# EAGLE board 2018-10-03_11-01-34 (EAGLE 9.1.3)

Size 160 x 100 mm. Coordinates in mm from the lower left corner, seen from the top.
Outline: 0,0 160,0 160,100 0,100 0,0
Copper layers (1*16): Top 0.035mm / dielectric 1.5mm / Bottom 0.035mm
Design rules "default": minimum track width 6mil, minimum drill 0.35mm, track to track 6mil, track to pad 6mil, pad to pad 6mil, via to via 6mil, smd to smd 6mil, copper to edge 40mil, drill to drill 6mil, minimum pad ring 10mil, minimum via ring 8mil, stop-mask expansion 4mil, vias tented up to drill 0mil, thermal gap 10mil

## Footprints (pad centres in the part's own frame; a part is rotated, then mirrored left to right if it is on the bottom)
0603 = drill 0: 1 -0.699,0; 2 0.699,0
1812 = drill 0: 1 -2.273,0; 2 2.273,0
CAPSMT_62_C10 = drill 0: 1 -2.273,0; 2 2.273,0
SM_RADIAL_J16 = drill 0: 1 -6.566,0; 2 6.566,0
1210_270 = drill 0: 1 -1.45,0; 2 1.45,0
0402 = drill 0: 1 -0.419,0; 2 0.419,0
SOD-323 = drill 0: 1 -1.1,0; 2 1.1,0
WB_GND = drill 0: 1 0,0
WB_CURRENT_LOAD = drill 0: 1 0,0; 2 0,0
MSS1210 = drill 0: 1 -4.763,0; 2 4.763,0
TRANS_NEXFET_Q5B = drill 0: 1 -2.77,1.905; 2 -2.77,0.635; 3 -2.77,-0.635; 4 -2.77,-1.905; 5 2.77,-1.905; 6 2.77,-0.635; 7 2.77,0.635; 8 2.77,1.905; 9 1.16,0
DNH0008A = drill 0: 1 -1.625,0.975; 2 -1.625,0.325; 3 -1.625,-0.325; 4 -1.625,-0.975; 5 1.385,-0.975; 6 1.385,-0.325; 7 1.385,0.325; 8 1.385,0.975; 9 0.205,0
0201 = drill 0: 1 -0.292,0; 2 0.292,0
2512 = drill 0: 1 -2.248,0; 2 2.248,0
1210 = drill 0: 1 -1.499,0; 2 1.499,0
MXA20A = drill 0: 1 -2.845,2.925; 2 -2.845,2.275; 3 -2.845,1.625; 4 -2.845,0.975; 5 -2.845,0.325; 6 -2.845,-0.325; 7 -2.845,-0.975; 8 -2.845,-1.625; 9 -2.845,-2.275; 10 -2.845,-2.925; 11 2.845,-2.925; 12 2.845,-2.275; 13 2.845,-1.625; 14 2.845,-0.975; 15 2.845,-0.325; 16 2.845,0.325; 17 2.845,0.975; 18 2.845,1.625; 19 2.845,2.275; 20 2.845,2.925; 21 0,0
WB_BATTERY = drill 0: 1 0,0; 2 0,0

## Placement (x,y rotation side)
CBST  330nF  [0603]  not placed on the board
CCOMP  27nF  [1812]  not placed on the board
CCOMP2  1.5nF  [0603]  not placed on the board
CIN  270uF  [CAPSMT_62_C10]  not placed on the board
COUT  470uF  [SM_RADIAL_J16]  not placed on the board
COUT_2  470uF  [SM_RADIAL_J16]  not placed on the board
COUT_3  470uF  [SM_RADIAL_J16]  not placed on the board
COUT_4  470uF  [SM_RADIAL_J16]  not placed on the board
COUTX  10uF  [1210_270]  not placed on the board
COUTX_2  10uF  [1210_270]  not placed on the board
COUTX_3  10uF  [1210_270]  not placed on the board
COUTX_4  10uF  [1210_270]  not placed on the board
CRES  470nF  [0603]  not placed on the board
CSS  220nF  [0402]  not placed on the board
CVCC  4.7uF  [0603]  not placed on the board
CVIN  470nF  [0603]  not placed on the board
DBST  540mV  [SOD-323]  not placed on the board
GND1  WB_GND  [WB_GND]  not placed on the board
GND2  WB_GND  [WB_GND]  not placed on the board
GND3  WB_GND  [WB_GND]  not placed on the board
GND4  WB_GND  [WB_GND]  not placed on the board
GND5  WB_GND  [WB_GND]  not placed on the board
IOUT  WB_CURRENT_LOAD  [WB_CURRENT_LOAD]  not placed on the board
L1  68uH  [MSS1210]  not placed on the board
M1  60V  [TRANS_NEXFET_Q5B]  not placed on the board
M2  60V  [DNH0008A]  not placed on the board
RCOMP  36.5k  [0201]  not placed on the board
RFBB  1.6k  [0603]  not placed on the board
RFBT  46.4k  [0402]  not placed on the board
RSENSE  4m  [2512]  not placed on the board
RSLOPE  301k  [0402]  not placed on the board
RT  162k  [0201]  not placed on the board
RUVB  8.25k  [0402]  not placed on the board
RUVT  51.1k  [0402]  not placed on the board
RVIN  2.74  [1210]  not placed on the board
U1  LM5122MH/NOPB  [MXA20A]  not placed on the board
VIN  WB_BATTERY  [WB_BATTERY]  not placed on the board

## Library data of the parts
CBST = AcceleratedDesigns_Lib; CAP: 3.3E-7; DATASHEET_URL: https://product.tdk.com/en/search/capacitor/ceramic/mlcc/info?part%5Fno%3DC1608X5R1H334K080AB; ESR: 0.016574; IRMS: 1.28367; MANUFACTURER_NAME: TDK; MANUFACTURER_PART_NUMBER: C1608X5R1H334K080AB; VDC: 50.0; VENDOR: TDK
CCOMP = AcceleratedDesigns_Lib; CAP: 2.7E-8; DATASHEET_URL: http://www.kemet.com/docfinder?Partnumber%3DC1812C273J5GACTU; ESR: 0.0; IRMS: 0.0; MANUFACTURER_NAME: Kemet; MANUFACTURER_PART_NUMBER: C1812C273J5GACTU; VDC: 50.0; VENDOR: Kemet
CCOMP2 = AcceleratedDesigns_Lib; CAP: 1.5E-9; DATASHEET_URL: http://www.murata.com/products/catalog/pdf/c03e.pdf; ESR: 0.0; IRMS: 0.0; MANUFACTURER_NAME: MuRata; MANUFACTURER_PART_NUMBER: GCM1885C1H152JA16D; VDC: 50.0; VENDOR: MuRata
CIN = AcceleratedDesigns_Lib; CAP: 2.7E-4; DATASHEET_URL: %20; ESR: 0.008; IRMS: 5.8; MANUFACTURER_NAME: Panasonic; MANUFACTURER_PART_NUMBER: 16SVPG270M; VDC: 16.0; VENDOR: Panasonic
COUT COUT_2-COUT_4 = AcceleratedDesigns_Lib; CAP: 4.7E-4; DATASHEET_URL: http://www.panasonic.com/industrial/components/pdf/smt%5Faec%5F050505.pdf; ESR: 0.082; IRMS: 1.41; MANUFACTURER_NAME: Panasonic; MANUFACTURER_PART_NUMBER: EEV-FK1J471M; VDC: 63.0; VENDOR: Panasonic
COUTX COUTX_2-COUTX_4 = AcceleratedDesigns_Lib; CAP: 1.0E-5; DATASHEET_URL: http://www.samsungsem.com/kr/support/product%2Dsearch/mlcc/%5F%5FicsFiles/afieldfile/2016/08/18/S%5FCL32B106KBJNNWE.pdf; ESR: 0.005; IRMS: 0.0; MANUFACTURER_NAME: Samsung Electro-Mechanics; MANUFACTURER_PART_NUMBER: CL32B106KBJNNWE; VDC: 50.0; VENDOR: Samsung Electro-Mechanics
CRES = AcceleratedDesigns_Lib; CAP: 4.7E-7; ESR: 0.0; IRMS: 0.0; MANUFACTURER_NAME: MuRata; MANUFACTURER_PART_NUMBER: GRM188R71E474KA12D; VDC: 25.0; VENDOR: MuRata
CSS = AcceleratedDesigns_Lib; CAP: 2.2E-7; ESR: 0.0; IRMS: 0.0; MANUFACTURER_NAME: MuRata; MANUFACTURER_PART_NUMBER: GRM155R61A224KE19D; VDC: 10.0; VENDOR: MuRata
CVCC = AcceleratedDesigns_Lib; CAP: 4.7E-6; DATASHEET_URL: https://product.tdk.com/en/search/capacitor/ceramic/mlcc/info?part%5Fno%3DC1608X6S1C475K080AC; ESR: 0.003728; IRMS: 2.69359; MANUFACTURER_NAME: TDK; MANUFACTURER_PART_NUMBER: C1608X6S1C475K080AC; VDC: 16.0; VENDOR: TDK
CVIN = AcceleratedDesigns_Lib; CAP: 4.7E-7; ESR: 0.0; IRMS: 0.0; MANUFACTURER_NAME: MuRata; MANUFACTURER_PART_NUMBER: GRM188R61C474KA93D; VDC: 16.0; VENDOR: MuRata
DBST = AcceleratedDesigns_Lib; DATASHEET_URL: http://www.torexsemi.com/products/schottky%5Fbarrier%5Fdiodes/data/XBS104S13.pdf; IO: 1.0; MANUFACTURER_NAME: Torex USA Corporation; MANUFACTURER_PART_NUMBER: XBS104S13R-G; VENDOR: Torex USA Corporation; VFATIO: 0.54; VRRM: 40.0
GND1-GND5 = AcceleratedDesigns_Lib; MANUFACTURER_NAME: WB_GND; MANUFACTURER_PART_NUMBER: WB_GND; POWERPORTTYPE: POWER_GROUND
IOUT = AcceleratedDesigns_Lib; MANUFACTURER_NAME: WB_CURRENT_LOAD; MANUFACTURER_PART_NUMBER: WB_CURRENT_LOAD; POWERPORTTYPE: POWER_GROUND
L1 = AcceleratedDesigns_Lib; DATASHEET_URL: http://www.coilcraft.com/pdfs/mss1210.pdf; DCR: 0.074; DESCRIPTION: Unknown; IDC: 4.3; L: 6.8E-5; MANUFACTURER: CoilCraft; MANUFACTURER_NAME: Coilcraft; MANUFACTURER_PART_NUMBER: MSS1210-683MEB; PACKAGE_DESIGNATOR: MSS1210; VENDOR: Coilcraft
M1 = AcceleratedDesigns_Lib; DATASHEET_URL: http://www.ti.com/lit/ds/symlink/csd18532q5b.pdf; IDSMAX: 100.0; MANUFACTURER_NAME: Texas Instruments; MANUFACTURER_PART_NUMBER: CSD18532Q5B; QGTYP: 21.0; QUANTITY: 1; RDSON45: 0.0043; VDSMAX: 60.0; VENDOR: Texas Instruments
M2 = AcceleratedDesigns_Lib; IDSMAX: 20.0; MANUFACTURER_NAME: Texas Instruments; MANUFACTURER_PART_NUMBER: CSD18543Q3A; QGTYP: 5.3; QUANTITY: 1; RDSON45: 0.0118; VDSMAX: 30.0; VENDOR: Texas Instruments
RCOMP = AcceleratedDesigns_Lib; DATASHEET_URL: http://www.yageo.com/documents/recent/PYu%2DRC%5FGroup%5F51%5FRoHS%5FL%5F5.pdf; MANUFACTURER_NAME: Yageo; MANUFACTURER_PART_NUMBER: RC0201FR-0736K5L; POWER: 0.05; RESISTANCE: 36500.0; TOLERANCE: 1.0; VENDOR: Yageo America
RFBB = AcceleratedDesigns_Lib; MANUFACTURER_NAME: Yageo; MANUFACTURER_PART_NUMBER: RC0603FR-071K6L; POWER: 0.1; RESISTANCE: 1600.0; TOLERANCE: 1.0; VENDOR: Yageo America
RFBT = AcceleratedDesigns_Lib; MANUFACTURER_NAME: Vishay-Dale; MANUFACTURER_PART_NUMBER: CRCW040246K4FKED; POWER: 0.063; RESISTANCE: 46400.0; TOLERANCE: 1.0; VENDOR: Vishay-Dale
RSENSE = AcceleratedDesigns_Lib; MANUFACTURER_NAME: Panasonic; MANUFACTURER_PART_NUMBER: ERJ-M1WSF4M0U; POWER: 1.0; RESISTANCE: 0.0040; TOLERANCE: 1.0; VENDOR: Panasonic
RSLOPE = AcceleratedDesigns_Lib; MANUFACTURER_NAME: Vishay-Dale; MANUFACTURER_PART_NUMBER: CRCW0402301KFKED; POWER: 0.063; RESISTANCE: 301000.0; TOLERANCE: 1.0; VENDOR: Vishay-Dale
RT = AcceleratedDesigns_Lib; DATASHEET_URL: http://www.yageo.com/documents/recent/PYu%2DRC%5FGroup%5F51%5FRoHS%5FL%5F5.pdf; MANUFACTURER_NAME: Yageo; MANUFACTURER_PART_NUMBER: RC0201FR-07162KL; POWER: 0.05; RESISTANCE: 162000.0; TOLERANCE: 1.0; VENDOR: Yageo America
RUVB = AcceleratedDesigns_Lib; MANUFACTURER_NAME: Vishay-Dale; MANUFACTURER_PART_NUMBER: CRCW04028K25FKED; POWER: 0.063; RESISTANCE: 8250.0; TOLERANCE: 1.0; VENDOR: Vishay-Dale
RUVT = AcceleratedDesigns_Lib; MANUFACTURER_NAME: Vishay-Dale; MANUFACTURER_PART_NUMBER: CRCW040251K1FKED; POWER: 0.063; RESISTANCE: 51100.0; TOLERANCE: 1.0; VENDOR: Vishay-Dale
RVIN = AcceleratedDesigns_Lib; DATASHEET_URL: http://www.yageo.com/documents/recent/PYu%2DRC1210%5F51%5FRoHS%5FL%5F%284%29.pdf; MANUFACTURER_NAME: Yageo; MANUFACTURER_PART_NUMBER: RC1210FR-072R74L; POWER: 0.5; RESISTANCE: 2.74; TOLERANCE: 1.0; VENDOR: Yageo
U1 = AcceleratedDesigns_Lib; DATASHEET_URL: http://www.ti.com/product/lm5122; FREQUENCY: 1000000.0; IMAX: 40.0; MANUFACTURER_NAME: Texas Instruments; MANUFACTURER_PART_NUMBER: LM5122MH/NOPB; MKTG_PACKAGE: MXA20A; NSID: LM5122MH/NOPB; PACKAGE: MXA20A; VENDOR: Texas Instruments
VIN = AcceleratedDesigns_Lib; MANUFACTURER_NAME: WB_BATTERY; MANUFACTURER_PART_NUMBER: WB_BATTERY; POWERPORTTYPE: POWER_GROUND

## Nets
0: CIN.2 COUT.2 COUT_2.2 COUT_3.2 COUT_4.2 COUTX.2 COUTX_2.2 COUTX_3.2 COUTX_4.2 CRES.2 CSS.2 CVCC.1 CVIN.2 GND1.1 GND2.1 GND3.1 GND4.1 GND5.1 IOUT.2 M1.1 M1.2 M1.3 RFBB.2 RSLOPE.2 RT.2 RUVB.2 U1.2 U1.9 U1.13 U1.15 U1.21 VIN.2
1: RUVB.1 RUVT.2 U1.6
2: CVIN.1 RVIN.2 U1.5
3: RSLOPE.1 U1.12
4: CIN.1 RSENSE.1 RUVT.1 RVIN.1 U1.4 VIN.1
5: L1.1 RSENSE.2 U1.3
6: RT.1 U1.8
7: CVCC.2 DBST.2 U1.17
8: CBST.1 DBST.1 U1.20
9: CSS.1 U1.7
10: CRES.1 U1.14
11: CCOMP2.1 CCOMP.1 RFBB.1 RFBT.2 U1.10
12: M2.4 U1.19
13: M1.4 U1.16
14: CCOMP2.2 RCOMP.1 U1.11
15: COUT.1 COUT_2.1 COUT_3.1 COUT_4.1 COUTX.1 COUTX_2.1 COUTX_3.1 COUTX_4.1 IOUT.1 M2.5 M2.6 M2.7 M2.8 M2.9 RFBT.1
16: CBST.2 L1.2 M1.5 M1.6 M1.7 M1.8 M1.9 M2.1 M2.2 M2.3 U1.18
37: CCOMP.2 RCOMP.2

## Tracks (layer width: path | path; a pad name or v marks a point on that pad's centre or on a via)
0  (31 unrouted)
1  (2 unrouted)
2  (2 unrouted)
3  (1 unrouted)
4  (5 unrouted)
5  (2 unrouted)
6  (1 unrouted)
7  (2 unrouted)
8  (2 unrouted)
9  (1 unrouted)
10  (1 unrouted)
11  (4 unrouted)
12  (1 unrouted)
13  (1 unrouted)
14  (2 unrouted)
15  (14 unrouted)
16  (10 unrouted)
37  (1 unrouted)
